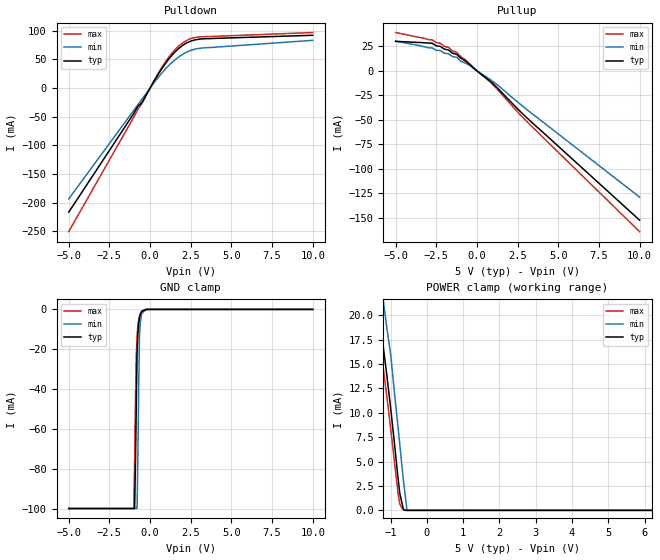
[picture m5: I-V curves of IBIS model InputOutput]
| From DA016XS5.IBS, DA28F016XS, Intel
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|**************************Input Output Model*********************************
[Model]   InputOutput
Model_type   I/O
|   for DQ[15:0]
Vinl = 0.8V
Vinh = 2.0V
| Variable   typ   min   max
C_comp   9.61p   NA   11.6p
[Voltage Range]   5.0V   4.5V   5.5V
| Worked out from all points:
|   slope of the pulldown table from 0 to 0.75 V, typ, clamps not added: 21.4 ohm
|   slope of the pullup table from 0 to 0.75 V, typ, clamps not added: 77.4 ohm
|   GND clamp passes 1 mA (typ) near -0.50 V on its own axis
|   POWER clamp passes 1 mA (typ) near -0.70 V on its own axis
[Pulldown]
| [Pullup] and [Pulldown] IV curves include only the current through
| the channels of output driver transistors when outputs are enabled
| with OE# = VIL.  Although the output driver transistors have np and
| pn diodes inherently created by CMOS IC fabrication between the
| drain and bulk of n-channel and p-channel CMOS transistors,
| the current through these junction diodes is not included in
| [Pullup] or [Pulldown].  Instead that drain/bulk diode current is
| included in the [POWER_clamp] or [GND_clamp] sections, which are
| not dependent on the state of OE# or output data value.
|Voltage  I(typ)   I(min)   I(max)
-5V       -216.7mA   -193.6mA   -250.7mA
-1V       -44.3mA    -38.76mA   -50.7mA
-750mV    -31.63mA   -29.09mA   -37.16mA
-500mV    -25.29mA   -19.32mA   -27.06mA
500mV     24.1mA     18.72mA    25.75mA
1V        45.14mA    35.08mA    48.15mA
1.25V     54.19mA    42.21mA    57.73mA
1.75V     68.98mA    54.19mA    73.15mA
2V        74.56mA    58.92mA    78.85mA
2.5V      82.03mA    65.74mA    86.62mA
3V        85.35mA    69.31mA    89.28mA
10V       92.2mA     83.4mA     97mA
[GND_clamp]
| [POWER_clamp] and [GND_clamp] IV curves describe ESD protection
| circuits PLUS some np and pn diodes which exist between the
| drain and bulk of n-channel and p-channel CMOS transistors.
| These drain/bulk diodes are inherent in CMOS IC fabrication,
| and are visible on the node of the I/O pin at all times.
| Even the drain/bulk diodes of output driver [Pullup] and [Powerdown]
| transistors are included in [POWER_clamp] or [GND_clamp], because
| these diodes contribute to I/O pin current even when the
| chip outputs are tristated by OE# = VIH.
| For example, when V forced on the I/O pin is large, we are
| forward biasing the pn diode at the drain/bulk interface in the
| p-channel pullup transistor.  Similarly, when V forced on the
| I/O pin is sufficiently negative with respect to the substrate
| ground, we are forward biasing the np diode at the drain/bulk
| interface in the n-channel pulldown transistor.  The effects
| of these diodes are included in [POWER_clamp] or [GND_clamp].
|Voltage  I(typ)   I(min)   I(max)
-5V       -99.95mA   -99.95mA   -99.95mA
-1V       -99.95mA   -99.95mA   -99.95mA
-950mV    -99.95mA   -99.95mA   -76.84mA
-900mV    -78.91mA   -99.95mA   -47.53mA
-850mV    -49.31mA   -99.95mA   -23.73mA
-800mV    -22.16mA   -99.95mA   -13.64mA
-750mV    -12.53mA   -74.6mA    -7.902mA
-700mV    -7.046mA   -39.88mA   -5.001mA
-650mV    -4.246mA   -12.75mA   -3.317mA
-600mV    -2.656mA   -6.915mA   -2.154mA
-500mV    -960uA     -1.953mA   -725.8uA
10V       0A         0A         0A
[Pullup]
| (Voltages for [Pullup] and [POWER_clamp] are specified with
| negative respect to Vcc.  Reference the IBIS documentation
| for more information regarding Vtable = Vcc - Voutput.
| This method keeps -Vds constant for the values in all three
| columns across a line of the table.
| [Pullup] and [Pulldown] IV curves include only the current through
| the channels of output driver transistors when outputs are enabled
| with OE# = VIL.  Although the output driver transistors have np and
| pn diodes inherently created by CMOS IC fabrication between the
| drain and bulk of n-channel and p-channel CMOS transistors,
| the current through these junction diodes is not included in
| [Pullup] or [Pulldown].  Instead that drain/bulk diode current is
| included in the [POWER_clamp] or [GND_clamp] sections, which are
| not dependent on the state of OE# or output data value.
|Voltage  I(typ)   I(min)   I(max)
-5V       30.1mA     30.4mA     39.1mA
-2.75V    28.19mA    23.37mA    31.58mA
-2.25V    24.99mA    20.65mA    28.16mA
-2V       22.12mA    18.02mA    24.95mA
-1.75V    21.33mA    17.5mA     23.96mA
-1.5V     17.93mA    14.51mA    20.28mA
-1.25V    16.93mA    13.94mA    18.99mA
-1V       13mA       9.96mA     14.61mA
-500mV    7.346mA    6.032mA    7.901mA
1V        -13.37mA   -11.02mA   -14.42mA
3V        -46.88mA   -38.63mA   -50.64mA
10V       -152.5mA   -129mA     -164.2mA
[POWER_clamp]
| (Voltages for [Pullup] and [POWER_clamp] are specified with
| negative respect to Vcc.  Reference the IBIS documentation
| for more information regarding Vtable = Vcc - Voutput.
| This method keeps -Vds constant for the values in all three
| columns across a line of the table.
| [POWER_clamp] and [GND_clamp] IV curves describe ESD protection
| circuits PLUS some np and pn diodes which exist between the
| drain and bulk of n-channel and p-channel CMOS transistors.
| These drain/bulk diodes are inherent in CMOS IC fabrication,
| and are visible on the node of the I/O pin at all times.
| Even the drain/bulk diodes of output driver [Pullup] and [Powerdown]
| transistors are included in [POWER_clamp] or [GND_clamp], because
| these diodes contribute to I/O pin current even when the
| chip outputs are tristated by OE# = VIH.
| For example, when V forced on the I/O pin is large, we are
| forward biasing the pn diode at the drain/bulk interface in the
| p-channel pullup transistor.  Similarly, when V forced on the
| I/O pin is sufficiently negative with respect to the substrate
| ground, we are forward biasing the np diode at the drain/bulk
| interface in the n-channel pulldown transistor.  The effects
| of these diodes are included in [POWER_clamp] or [GND_clamp].
|Voltage  I(typ)   I(min)   I(max)
-5V       99.99mA    99.99mA    99.98mA
-1.5V     24.8mA     29.32mA    22.56mA
-1.4V     22.2mA     26.8mA     19.95mA
-1.3V     19.49mA    24.18mA    17.25mA
-1.2V     16.67mA    21.45mA    14.45mA
-1.1V     13.69mA    18.57mA    11.52mA
-1V       10.49mA    16mA       8.396mA
-800mV    3.434mA    8.671mA    1.871mA
-750mV    1.778mA    6.81mA     668.2uA
-650mV    122.9uA    3.126mA    17.72uA
-550mV    0A         0A         0A
10V       0A         0A         0A
[Ramp]
| The DQ Ramp information is not provided at this time for the
| device but will be available in the future.  The table below
| is for the compatibility with some IBIS parsers.
| Variable   typ   min   max
 dV/dt_r   0V/0ns   0V/0ns   0V/0ns
 dV/dt_f   0V/0ns   0V/0ns   0V/0ns
